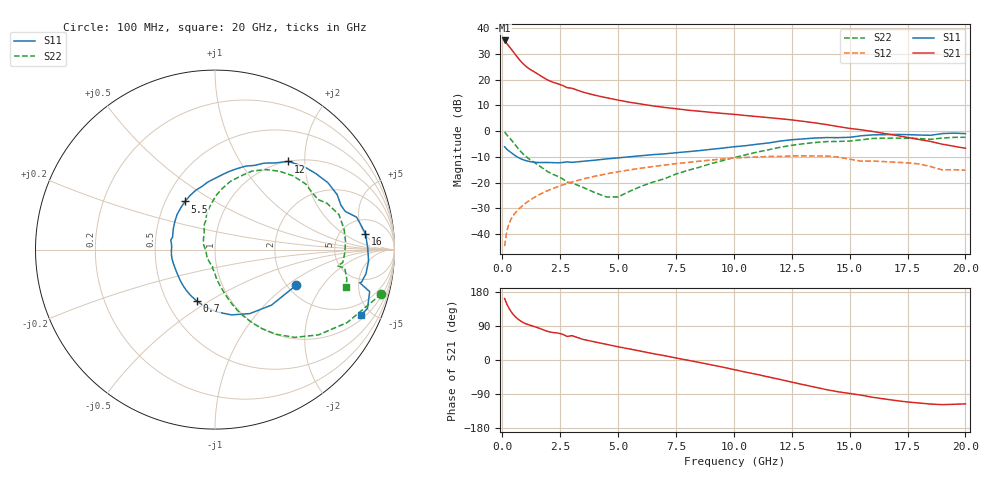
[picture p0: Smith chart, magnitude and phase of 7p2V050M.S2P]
! Infineon Technologies  Discrete & RF Semiconductors
! bfp620
! VCE =  2.0 V,  IC =  50 mA
! Common Emitter S-Parameters:  Sep 2002
# GHz  S  MA  R  50
!  f  S11  S21  S12  S22
! GHz  MAG  ANG  MAG  ANG  MAG  ANG  MAG  ANG
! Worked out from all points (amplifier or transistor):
!   59 points, 100 MHz to 20 GHz, reference 50 ohm
!   highest |S21| = 35.2 dB at 100 MHz (marker M1)
!   |S21| within 3 dB of that: start of sweep to 353 MHz
!   unconditionally stable (mu >= 1): 2.658 GHz to 9.834 GHz; 17.19 GHz to end of sweep
!   at 1 GHz: K = 0.85, MSG = 26.7 dB, |S12| = -28.1 dB
!   at 5.5 GHz: K = 1.04, MAG = 12.0 dB, |S12| = -15.1 dB
!   at 20 GHz: K = 1.26, MAG = 1.2 dB, |S12| = -15.2 dB
!   S11 on the Smith chart (normalised r, x): 100 MHz: 2.24, -1.17; 700 MHz: 0.70, -0.44; 5.5 GHz: 0.63, +0.37; 12 GHz: 1.00, +1.66; 16 GHz: 8.47, +5.25; 20 GHz: 1.22, -4.32
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0.1  0.4949 -23.5  57.5 162.3  0.0058 79.3  0.9594 -14.9
0.2  0.4413 -44.5  49.61 147.1  0.0116 73.0  0.8412 -28.9
0.3  0.4058 -61.5  43.6 135.2  0.0163 70.1  0.7469 -39.5
0.4  0.3752 -75.8  38.31 125.9  0.0203 68.1  0.6611 -47.7
0.5  0.3476 -88.3  33.5 118.4  0.0238 66.7  0.5817 -54.2
0.6  0.3238 -99.4  29.24 112.2  0.027 65.8  0.5106 -59.4
0.7  0.3045 -109.3  25.62 107.0  0.0302 65.1  0.4495 -63.6
0.8  0.2893 -117.9  22.65 102.6  0.0332 64.6  0.3988 -67.1
1  0.268 -131.5  18.45 96.1  0.0394 63.9  0.3255 -72.1
1.3  0.2505 -146.2  14.82 89.8  0.0488 62.8  0.2593 -76.8
1.8  0.2446 -166.1  10.79 78.9  0.0644 60.0  0.182 -84.4
2.8  0.2523 167.7  6.959 62.1  0.0958 52.3  0.1016 -98.5
3  0.2462 163.7  6.79 64.4  0.102 50.6  0.0986 -97.1
3.5  0.2587 154.1  5.671 54.1  0.1175 46.0  0.0801 -110.2
5.5  0.3161 122.0  3.625 29.1  0.1759 27.1  0.0676 158.4
7  0.3601 101.3  2.878 11.5  0.2182 12.6  0.1181 120.3
10.5  0.5187 64.8  2.005 -31.9  0.3073 -26.9  0.344 83.0
12  0.6387 50.3  1.735 -51.4  0.321 -44.6  0.4836 64.8
13.5  0.7312 30.6  1.441 -71.6  0.3275 -63.3  0.5982 43.4
16  0.8432 6.1  0.98 -98.4  0.2606 -87.3  0.7174 15.8
17  0.858 -4.3  0.826 -107.0  0.2479 -95.3  0.7289 3.6
20  0.8908 -24.3  0.463 -115.8  0.1734 -104.9  0.7568 -15.8
